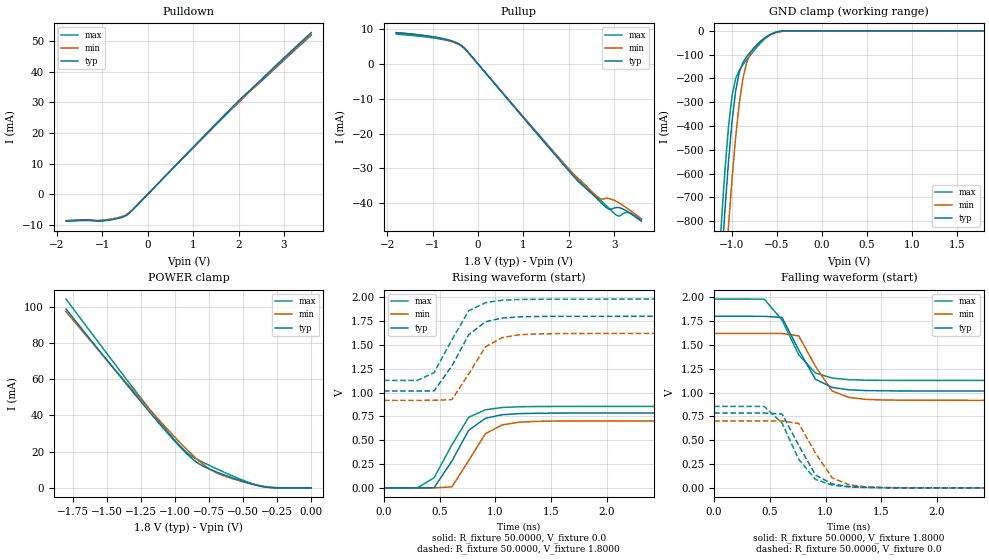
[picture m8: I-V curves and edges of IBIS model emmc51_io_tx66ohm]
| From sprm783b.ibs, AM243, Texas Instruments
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|   Model emmc51_io_tx66ohm
[Model]  emmc51_io_tx66ohm
Model_type I/O
Polarity   Non-Inverting
Enable   Active-High
Vinl =   0.6300V
Vinh =   1.1700V
Vmeas =  0.2000V
Cref =   0.5000pF
Rref =   50.0000
Vref =   0.2000V
C_comp   2.0000pF   2.0000pF   2.0000pF
[Temperature Range]   25.0000   0.1250k   -40.0000
[Voltage Range]   1.8000V   1.6200V   1.9800V
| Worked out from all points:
|   slope of the pulldown table from 0 to 0.27 V, typ, clamps not added: 64.7 ohm
|   slope of the pullup table from 0 to 0.27 V, typ, clamps not added: 64.4 ohm
|   GND clamp passes 1 mA (typ) near -0.43 V on its own axis
|   POWER clamp passes 1 mA (typ) near -0.38 V on its own axis
|   rising waveform, R_fixture 50.0000, V_fixture 0.0: 20-80 % time 250ps typ, 226ps min, 251ps max; typ from 0 V to 0.785 V
|   rising waveform, R_fixture 50.0000, V_fixture 1.8000: 20-80 % time 257ps typ, 228ps min, 245ps max; typ from 1.02 V to 1.8 V
|   falling waveform, R_fixture 50.0000, V_fixture 1.8000: 20-80 % time 220ps typ, 221ps min, 263ps max; typ from 1.8 V to 1.02 V
|   falling waveform, R_fixture 50.0000, V_fixture 0.0: 20-80 % time 223ps typ, 224ps min, 245ps max; typ from 0.785 V to 0 V
[Pulldown]
|Voltage   I(typ)   I(min)   I(max)
-1.8V     -8.87mA    -8.738mA   -8.632mA
-1.38V    -8.606mA   -8.481mA   -8.356mA
-1.14V    -8.826mA   -8.596mA   -8.648mA
-960mV    -8.714mA   -8.515mA   -8.479mA
-600mV    -7.729mA   -7.444mA   -7.594mA
-480mV    -7.014mA   -6.728mA   -6.947mA
-420mV    -6.385mA   -6.171mA   -6.317mA
-240mV    -3.713mA   -3.677mA   -3.648mA
1.62V     24.85mA    24.61mA    24.44mA
2.22V     33.6mA     33.2mA     33.29mA
3.6V      52.86mA    52.24mA    52mA
[Pullup]
|Voltage   I(typ)   I(min)   I(max)
-1.8V     8.936mA    8.977mA    8.523mA
-840mV    7.444mA    7.329mA    7.141mA
-360mV    5.265mA    5.024mA    5.198mA
-180mV    2.794mA    2.755mA    2.744mA
1.92V     -29.46mA   -29.1mA    -28.97mA
2.4V      -35.94mA   -35.26mA   -35.96mA
2.7V      -39.67mA   -38.75mA   -39.1mA
2.88V     -41.66mA   -38.6mA    -41.35mA
3.06V     -41.19mA   -39.53mA   -43.5mA
3.12V     -41.28mA   -40mA      -43.68mA
3.3V      -42.43mA   -41.58mA   -42.64mA
3.6V      -45.17mA   -44.43mA   -44.76mA
[GND_clamp]
|Voltage   I(typ)   I(min)   I(max)
-1.8V     -6.702A    -6.906A    -6.586A
-1.12V    -991.1mA   -1.287A    -813.9mA
-1.08V    -758.6mA   -1.044A    -591.9mA
-1.04V    -552.1mA   -821.7mA   -405.1mA
-1V       -379.5mA   -621.1mA   -272.1mA
-960mV    -252.2mA   -446.8mA   -200.8mA
-920mV    -175.1mA   -305.6mA   -166.2mA
-880mV    -134mA     -202.7mA   -143.1mA
-800mV    -90.55mA   -97.27mA   -103.4mA
-600mV    -20.52mA   -21.87mA   -22.63mA
-400mV    -332.1uA   -1.109mA   -151.2uA
1.8V      231.4nA    26.73uA    254.2nA
[POWER_clamp]
|Voltage   I(typ)   I(min)   I(max)
-1.8V     98.61mA    97.2mA     104.1mA
-1.44V    64.88mA    65.13mA    68.09mA
-1.16V    39.38mA    40.99mA    40.81mA
-1V       25.58mA    27.85mA    26.18mA
-900mV    17.84mA    20.17mA    18.67mA
-820mV    13.08mA    14.63mA    15mA
-740mV    10.1mA     10.15mA    12.1mA
-660mV    7.73mA     7.169mA    9.318mA
-560mV    4.993mA    4.669mA    6.008mA
-440mV    2.128mA    2.259mA    2.491mA
-340mV    491.7uA    786.4uA    470uA
0V        231.4nA    1.21uA     740.9nA
[Ramp]
| variable   typ   min   max
dV/dt_r  0.4710/0.2460n   0.4214/0.2260n   0.5128/0.2427n
dV/dt_f  0.4701/0.2202n   0.4210/0.2212n   0.5119/0.2604n
R_load = 50.0000
[Rising Waveform]
R_fixture= 50.0000
V_fixture= 0.0
V_fixture_min= 0.0
V_fixture_max= 0.0
|time   V(typ)   V(min)   V(max)
0s        1.74uV     17.69uV    3.633uV
300ps     127.6uV    35.3uV     441.2uV
450ps     976.8uV    270.8uV    105.7mV
610ps     281.4mV    10.44mV    451.2mV
760ps     603.2mV    285.9mV    739.4mV
910ps     729.7mV    567.9mV    818.8mV
1.06ns    766.9mV    660.4mV    843mV
1.36ns    782.7mV    697.2mV    853.2mV
1.82ns    784.9mV    702mV      854.6mV
15ns      785.1mV    702.4mV    854.7mV
[Rising Waveform]
R_fixture= 50.0000
V_fixture= 1.8000
V_fixture_min= 1.6200
V_fixture_max= 1.9800
|time   V(typ)   V(min)   V(max)
0s        1.016V     918.3mV    1.127V
300ps     1.017V     918.3mV    1.127V
450ps     1.018V     918.6mV    1.209V
610ps     1.28V      925.9mV    1.553V
760ps     1.605V     1.194V     1.857V
910ps     1.742V     1.478V     1.942V
1.06ns    1.781V     1.577V     1.968V
1.21ns    1.794V     1.606V     1.976V
1.67ns    1.8V       1.619V     1.98V
15ns      1.8V       1.62V      1.98V
[Falling Waveform]
R_fixture= 50.0000
V_fixture= 1.8000
V_fixture_min= 1.6200
V_fixture_max= 1.9800
|time   V(typ)   V(min)   V(max)
0s        1.8V       1.62V      1.98V
450ps     1.8V       1.62V      1.98V
610ps     1.788V     1.62V      1.76V
760ps     1.445V     1.594V     1.395V
910ps     1.139V     1.275V     1.205V
1.06ns    1.054V     1.016V     1.152V
1.21ns    1.029V     948.6mV    1.135V
1.52ns    1.018V     922.1mV    1.128V
1.97ns    1.017V     918.6mV    1.127V
15ns      1.016V     918.3mV    1.127V
[Falling Waveform]
R_fixture= 50.0000
V_fixture= 0.0
V_fixture_min= 0.0
V_fixture_max= 0.0
|time   V(typ)   V(min)   V(max)
0s        785.1mV    702.4mV    854.7mV
450ps     784.9mV    702.3mV    854.2mV
610ps     774.8mV    702.1mV    679.7mV
760ps     445.4mV    675.5mV    298.9mV
910ps     134.9mV    364.3mV    88.41mV
1.06ns    41.84mV    104.1mV    28.5mV
1.21ns    13.87mV    33.01mV    9.627mV
1.52ns    1.919mV    4.286mV    1.204mV
1.97ns    133.6uV    343uV      74.36uV
15ns      1.706uV    17.63uV    3.581uV
